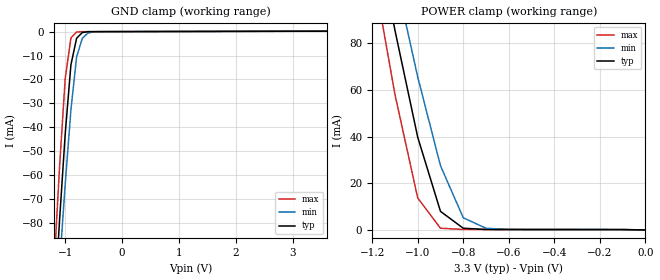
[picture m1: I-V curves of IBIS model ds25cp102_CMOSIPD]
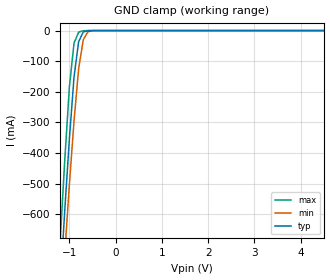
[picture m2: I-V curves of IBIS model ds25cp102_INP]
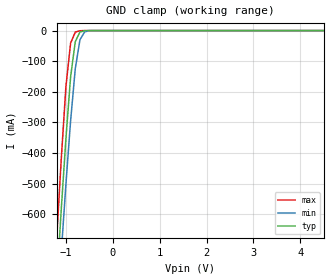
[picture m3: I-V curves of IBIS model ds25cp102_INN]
|   National Semiconductor Corporation
|   IBIS Model
|   of
|   ds25cp102
|  (no equalization, no pre-emphasis)
[IBIS Ver]   3.2
[Comment Char]   |_char
[File name]   ds25cp102.ibs
[File Rev]   1.0
[Date]   11/28/2007
[Source]
[Notes]
Rev 1.0   First release.
NOTICE:   The nature of the pre-emphasis and equalization circuitry
   precludes them from being properly modeled by the simple
   I/V and V/T data in the IBIS model.  Therefore, this model
   is only valid for this device when EQ and PE pins are set
   to logic 0.
[Disclaimer]
(C) Copyright National Semiconductor Corporation 2005
   All rights reserved
   National Semiconductor Corporation hereby grants
the user of this IBIS model a non-exclusive, nontransferable
license to use this IBIS model under the following terms.
Before using this IBIS model, the user should read this
license.  If the user does not accept these terms,  the
IBIS model should be returned to National within 30 days.
   The user is granted this license only to use the
IBIS model and is not granted rights to sell, load, rent,
lease or license the IBIS model in whole or in part, or in
modified form to anyone other than user. User may modify
the IBIS model to suit its specific applications but rights
to derivative works and such modifications shall belong to
National.
   This IBIS model is provided on an "AS IS" basis and
National makes absolutely no warranty with respect to the
information contained herein.NATIONAL DISCLAIMS AND CUSTOMER
WAIVES ALL WARRANTIES, EXPRESS OR IMPLIED, INCLUDING
WARRANTIES OF MERCHANTABILITY OR FITNESS FOR A PARTICULAR
PURPOSE. The entire risk as to quality and performance is
with the Customer. ACCORDINGLY, IN NO EVENT SHALL THE
COMPANY BE LIABLE FOR ANY DAMAGES, WHETHER IN CONTRACT OR
TORT,INCLUDING ANY LOST PROFITS OR OTHER INCIDENTAL,
CONSEQUENTIAL, EXEMPLARY, OR PUNITIVE DAMAGES ARISING OUT
OF THE USE OR APPLICATION OF THE IBIS model provided in
this package.Further, National reserves the right to make
changes without notice to any product herein to improve
reliability, function, or design. National does not convey
any license under patent rights or any other intellectual
property rights, including those of third parties.
   National is not obligated to provide maintenance or support
for the licensed IBIS model.
Contact National at ATTN:INTERFACE/IBIS MODELS.
5 Foden Road, M/S 01-50, South Porltand, ME 04106
(207) 541-8467
[Copyright]
(c) Copyright 2005 National Semiconductor Corp.
[Component]   ds25cp102
Si_location Pin
Timing_location Pin
[Manufacturer]   National Semiconductor Corp.
[Package]
|   TYP   MIN   MAX
R_pkg   58m   53m   66m
L_pkg   0.717n   0.629n   0.858n
C_pkg   0.053p   0.042p   0.069p
[Pin]   signal_name   model_name   R_pin   L_pin   C_pin
1   IN0+   ds25cp102_INP   0.053 0.629n  0.061p
2   IN0-   ds25cp102_INN   0.055 0.673n  0.042p
3   IN1+   ds25cp102_INP   0.055 0.664n  0.042p
4   IN1-   ds25cp102_INN   0.053 0.629n  0.059p
5   GND   GND   0.064 0.845n  0.068p
6   EQ   ds25cp102_CMOSIPD   0.065 0.857n  0.043p
7   SEL0   ds25cp102_CMOSIPD   0.066 0.857n  0.042p
8   SEL1   ds25cp102_CMOSIPD   0.060 0.76n   0.068p
9   OUT1-   ds25cp102_OUTN   0.053 0.638n  0.059p
10   OUT1+   ds25cp102_OUTP   0.054 0.653n  0.042p
11   OUT0-   ds25cp102_OUTN   0.055 0.668n  0.042p
12   OUT0+   ds25cp102_OUTP   0.053 0.634n  0.06p
13   EN1   ds25cp102_CMOSIPD   0.060 0.747n  0.061p
14   EN0   ds25cp102_CMOSIPD   0.059 0.725n  0.045p
15   PE   ds25cp102_CMOSIPD   0.060 0.736n  0.045p
16   VCC   POWER   0.059 0.741n  0.062p
[Series Pin Mapping]  pin_2   model_name
1   2   input_term
3   4   input_term
[Diff Pin] inv_pin  vdiff   tdelay_typ   tdelay_min   tdelay_max
| Receiver Vth = +/-100mV
1   2   0.10   0   0   0
3   4   0.10   0   0   0
10   9   0.00   0   0   0
12   11   0.00   0   0   0
|   Model input termination resistor
[Model]   input_term
Model_type   Series
Polarity   Non-Inverting
C_comp   0.0pF   0.0pF   0.0pF
[Temperature Range] 25   85   -40
[Voltage Range]   3.3   3.0   3.6
| Resistance   ohm(typ)   ohm(min)   ohm(max)
[R Series]   100   85   115
| Models and submodels in the file (6): ds25cp102_CMOSIPD (Input), ds25cp102_INP (Input), ds25cp102_INN (Input), ds25cp102_OUTP (Output), ds25cp102_OUTN (Output), input_term (Series)
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[Model]   ds25cp102_CMOSIPD
Model_type Input
Polarity Non-Inverting
Vinh=2.0
Vinl=0.8
C_comp   2pF   2pF   2pF
[Model Spec]
S_overshoot_high   3.3   3.0   3.6
S_overshoot_low   0.0   0.0   0.0
[Temperature Range]   25   85   -40
[Voltage Range]   3.3   3.0   3.6
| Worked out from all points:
|   GND clamp passes 1 mA (typ) near -0.73 V on its own axis
|   POWER clamp passes 1 mA (typ) near -0.80 V on its own axis
[GND Clamp]
-3.6V     -1.142A    -1.066A    -1.245A
-1.2V     -118.2mA   -134.1mA   -99.89mA
-1.1V     -79.12mA   -98.1mA    -56.83mA
-1V       -42.72mA   -63.75mA   -19.57mA
-900mV    -13.92mA   -32.77mA   -2.672mA
-800mV    -2.785mA   -10.65mA   -180.3uA
-700mV    -387.7uA   -2.808mA   -33.41uA
-600mV    -41.54uA   -587.4uA   -27.59uA
-500mV    -25.24uA   -68.41uA   -22.98uA
3.6V      180uA      222.2uA    165.5uA
[POWER Clamp]
-3.6V     1.477A     1.382A     1.606A
-1.2V     136mA      156.4mA    113.1mA
-1.1V     85.55mA    109.6mA    58.08mA
-1V       39.73mA    65.52mA    13.7mA
-900mV    7.959mA    27.51mA    750.9uA
-800mV    744.1uA    5.23mA     208.6uA
-700mV    217.4uA    717.8uA    197.7uA
-600mV    195.4uA    222.2uA    193.1uA
0V        -1.65nA    -1.598nA   -1.655nA
[Model]   ds25cp102_INP
Model_type Input
Polarity Non-Inverting
Vinh=1.25
Vinl=1.15
C_comp   1.7pF   1.7pF   1.7pF
[Model Spec]
S_overshoot_high   3.3   3.0   3.6
S_overshoot_low   0.0   0.0   0.0
[Temperature Range]   25   85   -40
[Voltage Range]   3.3   3.0   3.6
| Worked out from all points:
|   GND clamp passes 1 mA (typ) near -0.62 V on its own axis
[GND Clamp]
|V(groundclamp)   I(typ)   I(min)   I(max)
-3.6V     -7.949A    -7.688A    -8.364A
-1.2V     -837.2mA   -968.2mA   -688.4mA
-1.1V     -586.8mA   -729.1mA   -422.6mA
-1V       -353.4mA   -502.6mA   -183.7mA
-900mV    -151.8mA   -295.7mA   -40.94mA
-800mV    -36.07mA   -124.3mA   -4.991mA
-700mV    -4.641mA   -29.98mA   -506.7uA
-600mV    -299.4uA   -4.1mA     -51.64uA
-500mV    -23.36uA   -273.5uA   -3.241uA
7.2V      407.9pA    9.955nA    116.1pA
[Model]   ds25cp102_INN
Model_type Input
Polarity Inverting
Vinh=1.25
Vinl=1.15
C_comp   1.7pF   1.7pF   1.7pF
[Model Spec]
S_overshoot_high   3.3   3.0   3.6
S_overshoot_low   0.0   0.0   0.0
[Temperature Range]   25   85   -40
[Voltage Range]   3.3   3.0   3.6
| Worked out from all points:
|   GND clamp passes 1 mA (typ) near -0.62 V on its own axis
[GND Clamp]
|V(groundclamp)   I(typ)   I(min)   I(max)
-3.6V     -7.949A    -7.688A    -8.364A
-1.2V     -837.2mA   -968.2mA   -688.4mA
-1.1V     -586.8mA   -729.1mA   -422.6mA
-1V       -353.4mA   -502.6mA   -183.7mA
-900mV    -151.8mA   -295.7mA   -40.94mA
-800mV    -36.07mA   -124.3mA   -4.991mA
-700mV    -4.641mA   -29.98mA   -506.7uA
-600mV    -299.4uA   -4.1mA     -51.64uA
-500mV    -23.36uA   -273.5uA   -3.241uA
7.2V      407.9pA    9.955nA    116.1pA
